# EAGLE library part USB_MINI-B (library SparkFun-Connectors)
USB type Mini-B Connector Breaks out 5th pin, and includes shield pins if needed. SparkFun Products: SparkFun FTDI Basic Breakout SparkFun XBee Explorer USB SparkFun Redboard
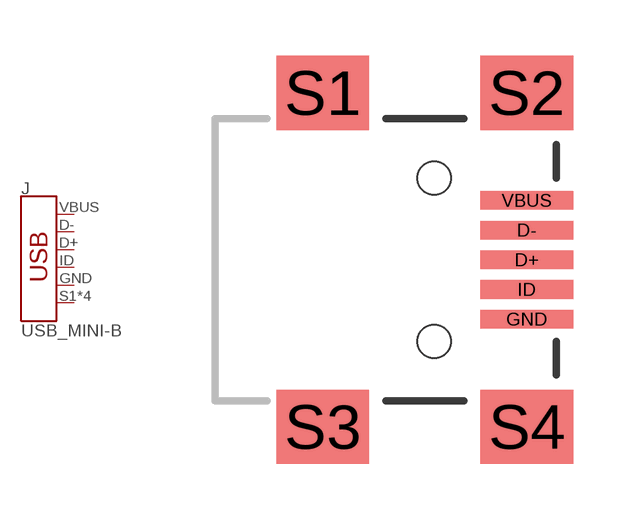
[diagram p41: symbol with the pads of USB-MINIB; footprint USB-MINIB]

Designator prefix J

## USB_MINI-B_SMT (PROD_ID: CONN-08193; SF_ID: PRT-00587)  [USB-MINIB]
D+  D+
D-  D-
GND  GND  pwr
ID  ID
S1  SHIELD
S2  SHIELD
S3  SHIELD
S4  SHIELD
VBUS  VBUS  pwr

## Footprint USB-MINIB (pad centres in mm)
USB Type Mini-B Surface Mounted Specifications: Pin count: 5 main, 4 shield pins Datasheet referenced for footprint Example device(s): USB_Mini-B
smd 2.5 x 0.5: D+ 2.5,0; D- 2.5,0.8; GND 2.5,-1.6; ID 2.5,-0.8; VBUS 2.5,1.6
smd 2.5 x 2: S1 -3,4.5; S2 2.5,4.5; S3 -3,-4.5; S4 2.5,-4.5
hole 0.9 at 0,2.2
hole 0.9 at 0,-2.2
